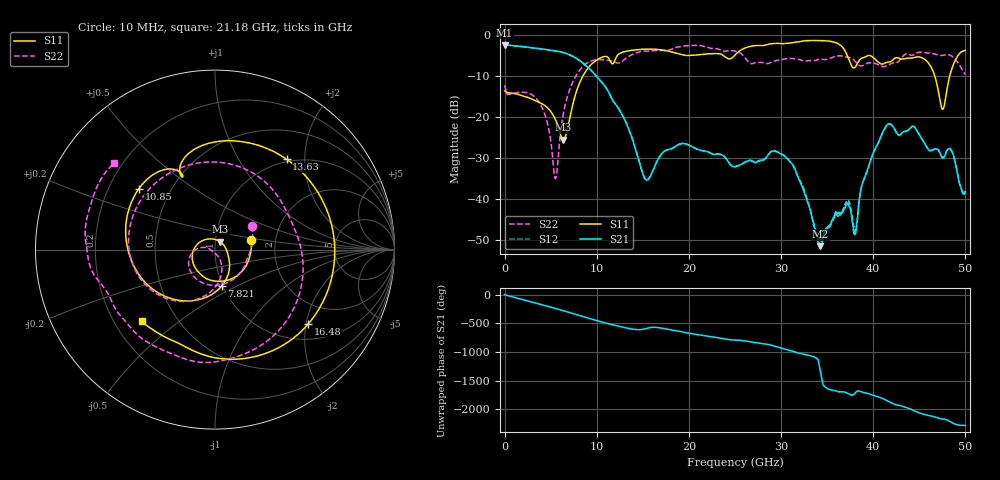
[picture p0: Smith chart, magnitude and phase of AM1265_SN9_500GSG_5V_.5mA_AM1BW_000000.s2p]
!Keysight Technologies,N5245B,MY58422270,A.16.20.02
!Date: Thursday, March 05, 2026 00:23:34
!Correction: S11(C  2-Port  )
!S21(C  2-Port  )
!S12(C  2-Port  )
!S22(C  2-Port  )
!S2P File: Measurements: S11, S21, S12, S22:
# Hz S  dB  R 50
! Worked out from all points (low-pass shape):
!   3201 points, 10 MHz to 50 GHz, reference 50 ohm
!   highest |S21| = -2.48 dB at 10 MHz (marker M1); lowest = -51.6 dB at 34.25 GHz (marker M2)
!   |S21| within 3 dB of the highest: start of sweep to 7.584 GHz
!   lowest |S11| = -25.6 dB at 6.368 GHz (marker M3), VSWR 1.11, Z = 52.8 + j4.61 ohm
!   |S11| at or under -10 dB: start of sweep to 8.52 GHz; 46.67 GHz to 48.3 GHz (1.635 GHz wide, 3.44 % of centre)
!   |S22| runs from -35.1 to -2.5 dB; largest |S21 - S12| = 0.0087
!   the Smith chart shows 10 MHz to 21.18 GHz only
!   S11 on the Smith chart (normalised r, x): 10 MHz: 1.49, +0.16; 7.821 GHz: 0.99, -0.42; 10.85 GHz: 0.33, +0.32; 13.63 GHz: 0.96, +1.64; 16.48 GHz: 1.40, -2.06; 21.18 GHz: 0.31, -0.37
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1e7  -13.65 14.3  -2.48 4.2  -2.57 3.9  -12.32 32.4
1.931491e9  -14.88 -78.1  -2.88 -82.7  -2.88 -82.7  -14.02 -95.2
3.884225e9  -16.64 -141.9  -3.40 -165.8  -3.41 -165.7  -16.94 -165.8
5.5089e9  -20.61 152.4  -3.92 122.5  -3.93 122.5  -35.11 -133.2
6.368103e9  -25.62 56.3  -4.34 82.5  -4.35 82.5  -19.41 -69.1
7.820938e9  -13.69 -79.8  -5.80 12.4  -5.80 12.4  -9.76 -117.8
8.352081e9  -10.73 -107.3  -6.64 -13.3  -6.63 -13.2  -8.08 -138.2
1.085158e10  -5.30 141.2  -12.42 -128.0  -12.42 -128.0  -6.13 111.1
1.363228e10  -3.84 51.5  -23.91 127.8  -23.92 127.9  -5.07 -42.5
1.528819e10  -3.51 -2.8  -35.27 128.8  -35.32 129.0  -4.01 -107.9
1.647546e10  -3.55 -38.4  -31.20 151.6  -31.10 151.7  -3.87 -136.6
1.667854e10  -3.59 -44.2  -30.33 147.3  -30.22 147.7  -3.88 -140.7
2.117764e10  -4.85 -135.6  -28.16 19.4  -28.15 19.8  -2.60 139.6
2.5005e10  -4.96 175.0  -32.22 -66.3  -32.21 -67.0  -3.96 71.2
3.028519e10  -2.16 84.4  -29.41 139.1  -29.41 139.9  -5.94 -42.8
3.334708e10  -1.40 35.6  -44.41 9.1  -44.43 1.5  -6.32 -126.2
3.425315e10  -1.38 19.8  -51.61 124.4  -49.76 -66.6  -5.97 -144.7
3.808051e10  -7.79 -24.9  -48.54 94.4  -48.07 -132.2  -6.60 140.0
4.167354e10  -6.67 -53.5  -21.72 -59.5  -21.78 -60.0  -7.34 117.6
4.511035e10  -5.47 -100.6  -24.82 93.9  -24.87 93.8  -4.24 75.7
4.770358e10  -17.34 68.4  -29.82 -8.7  -29.66 -7.6  -4.95 39.5
5e10  -3.80 -71.1  -38.35 -117.9  -38.73 -125.8  -9.67 2.1
